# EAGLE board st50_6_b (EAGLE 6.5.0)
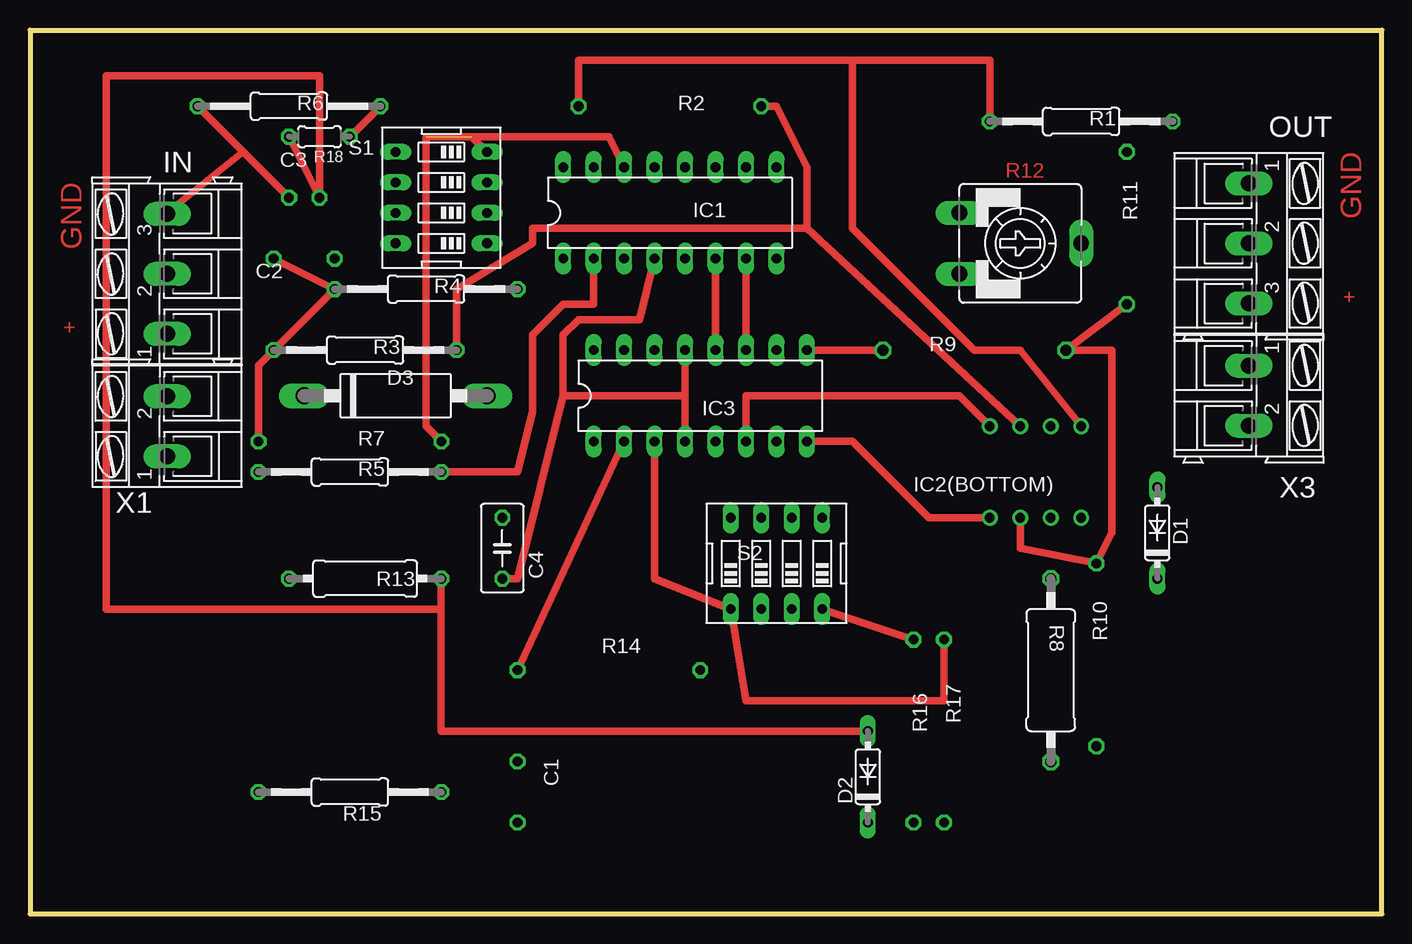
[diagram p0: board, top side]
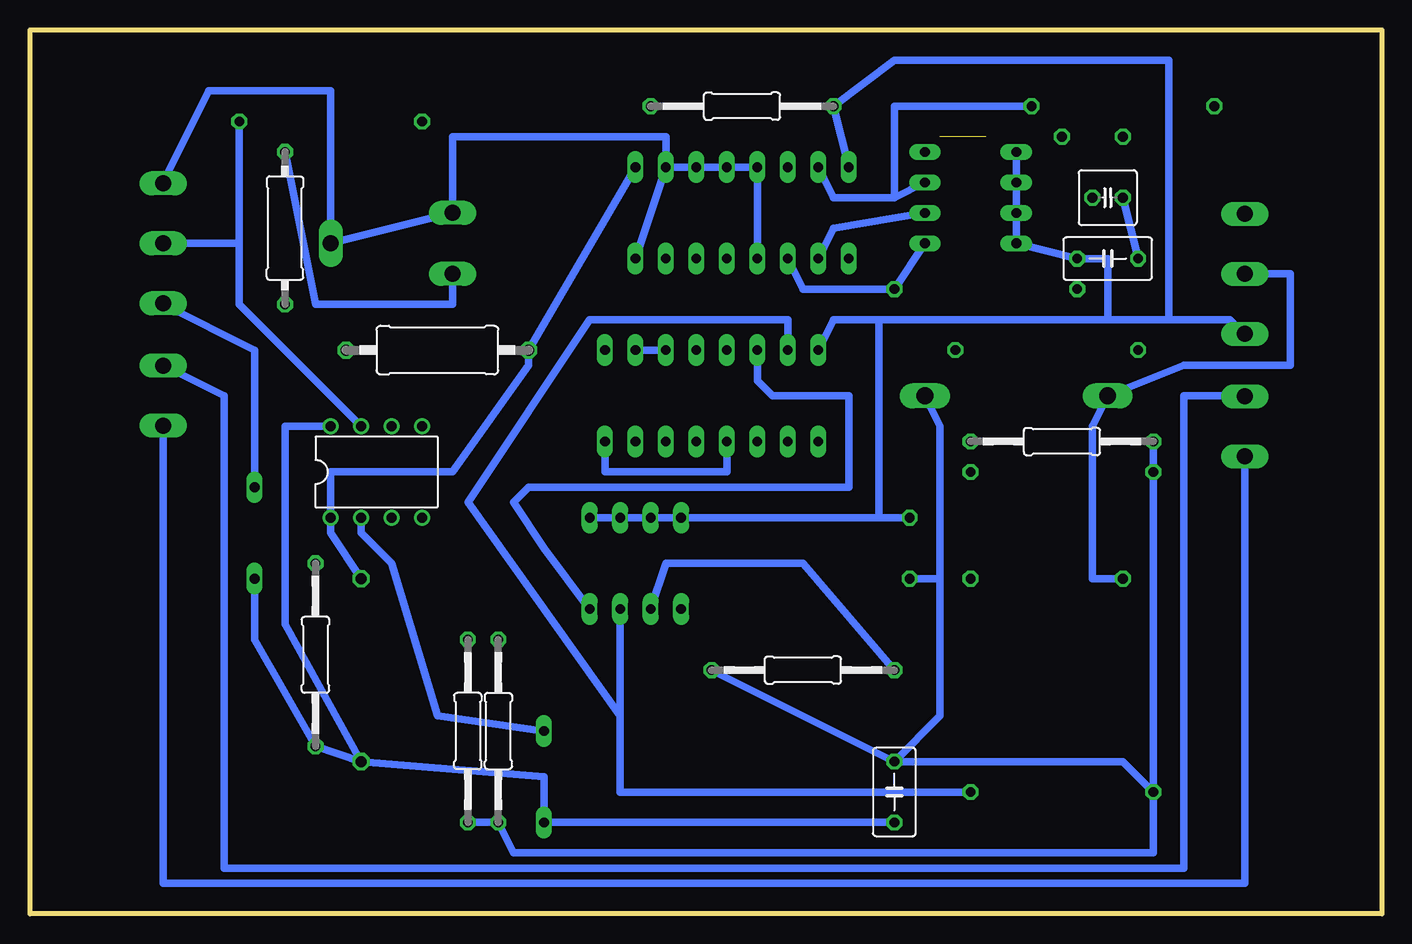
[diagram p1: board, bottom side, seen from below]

Size 112.7 x 73.66 mm. Coordinates in mm from the lower left corner, seen from the top.
Outline: 112.7,73.65 112.7,0 0,0 0,73.65
Outline: 0,73.66 112.7,73.66
Copper layers (1*16): Top 0.035mm / dielectric 1.5mm / Bottom 0.035mm
Design rules "ST50_4 *": minimum track width 0.4mm, minimum drill 24mil, track to track 0.4mm, track to pad 0.4mm, pad to pad 0.4mm, via to via 0.4mm, smd to smd 8mil, copper to edge 40mil, drill to drill 8mil, minimum pad ring 10mil, minimum via ring 8mil, stop-mask expansion 4mil, vias tented up to drill 0mil, thermal gap 10mil
Net classes: 0 default: clearance 0.355 mm

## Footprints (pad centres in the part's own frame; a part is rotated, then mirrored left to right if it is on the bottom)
C050-035X075 = drill 0.813 octagon: 1 -2.54,0; 2 2.54,0
C025-050X050 = drill 0.813 octagon: 1 -1.27,0; 2 1.27,0
DO35-7 = drill 0.813 long: A 3.81,0; C -3.81,0
C1702-15 = drill 1.397 long: A 7.62,0; C -7.62,0
DIL16 = drill 0.813 long: 1 -8.89,-3.81; 2 -6.35,-3.81; 3 -3.81,-3.81; 4 -1.27,-3.81; 5 1.27,-3.81; 6 3.81,-3.81; 7 6.35,-3.81; 8 8.89,-3.81; 9 8.89,3.81; 10 6.35,3.81; 11 3.81,3.81; 12 1.27,3.81; 13 -1.27,3.81; 14 -3.81,3.81; 15 -6.35,3.81; 16 -8.89,3.81
DIL08 = drill 0.813 pad 1.27: 1 -3.81,-3.81; 2 -1.27,-3.81; 3 1.27,-3.81; 4 3.81,-3.81; 5 3.81,3.81; 6 1.27,3.81; 7 -1.27,3.81; 8 -3.81,3.81
AK300/3 = drill 1.321 long: 1 -5.004,0; 2 0,0; 3 5.004,0
0207/15 = drill 0.813 octagon: 1 -7.62,0; 2 7.62,0
0411/15 = drill 0.914 octagon: 1 -7.62,0; 2 7.62,0
0309/12 = drill 0.813 octagon: 1 -6.35,0; 2 6.35,0
CA9V = drill 1.321 long: A -2.54,-5.08; E 2.54,-5.08; S 0,5.08
0204/5 = drill 0.813 octagon: 1 -2.54,0; 2 2.54,0
EDG-04 = drill 0.813 long: 1 -3.81,-3.81; 2 -1.27,-3.81; 3 1.27,-3.81; 4 3.81,-3.81; 5 3.81,3.81; 6 1.27,3.81; 7 -1.27,3.81; 8 -3.81,3.81
AK300/2 = drill 1.321 long: 1 -2.515,0; 2 2.489,0

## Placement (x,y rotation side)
C1  100nF  [C050-035X075]  40.64,10.16 90 bottom
C2  1µF 16V  [C050-035X075]  22.86,54.61 0 bottom
C3  10nF 50V  [C025-050X050]  22.86,59.69 0 bottom
C4  1µF 16V  [C050-035X075]  39.37,30.48 270 top
D1  1N4148DO35-7  [DO35-7]  93.98,31.75 90 top
D2  1N4148DO35-7  [DO35-7]  69.85,11.43 90 top
D3  1N5340  [C1702-15]  30.48,43.18 0 top
IC1  4089N  [DIL16]  53.34,58.42 0 top
IC2(BOTTOM)  LM393N  [DIL08]  83.82,36.83 0 bottom
IC3  4089N  [DIL16]  55.88,43.18 0 top
IN  IN  [AK300/3]  11.43,53.34 90 top
OUT  [AK300/3]  101.6,55.88 270 top
R1  10k  [0207/15]  87.63,66.04 0 top
R2  10k  [0207/15]  53.34,67.31 0 bottom
R3  10k  [0207/15]  27.94,46.99 0 top
R4  10k  [0207/15]  33.02,52.07 0 top
R5  10k  [0207/15]  26.67,36.83 0 top
R6  10k  [0207/15]  21.59,67.31 0 top
R7  10k  [0207/15]  26.67,39.37 0 bottom
R8  4.7k  [0411/15]  85.09,20.32 270 top
R9  1M  [0411/15]  78.74,46.99 0 bottom
R10  10k  [0207/15]  88.9,21.59 90 bottom
R11  1k  [0309/12]  91.44,57.15 270 bottom
R12  10k  [CA9V]  82.55,55.88 270 top
R13  22k  [0309/12]  27.94,27.94 0 top
R14  10k  [0207/15]  48.26,20.32 0 bottom
R15  10k  [0207/15]  26.67,10.16 0 top
R16  10k  [0207/15]  73.66,15.24 270 bottom
R17  10k  [0207/15]  76.2,15.24 90 bottom
R18  2M  [0204/5]  24.13,64.77 180 top
S1  Dip 4  [EDG-04]  34.29,59.69 90 top
S2  Dip 4  [EDG-04]  62.23,29.21 0 top
X1  [AK300/2]  11.43,40.64 90 top
X3  [AK300/2]  101.6,43.18 270 top

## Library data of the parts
C1-C4 R1-R11 R13-R18 = rcl
D1-D3 = diode
IC1 IC3 = 40xx
IC2(BOTTOM) = linear
IN OUT X1 X3 = con-ptr500; OC_FARNELL: unknown; OC_NEWARK: unknown
R12 = pot
S1 S2 = special

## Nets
+8V: C1.1 C2.1 C4.1 D1.C D2.C IC1.16 IC2(BOTTOM).8 IC3.16 IN.1 R1.1 R2.2 R8.2 R10.1 S1.5 S1.6 S1.7 S1.8 S2.5 S2.6 S2.7 S2.8
GND: C1.2 C2.2 C3.2 C4.2 D3.A IC1.4 IC1.8 IC1.10 IC1.11 IC1.12 IC1.13 IC2(BOTTOM).4 IC3.4 IC3.8 IC3.13 IN.3 OUT.1 R3.1 R4.1 R5.1 R6.1 R7.2 R12.A R12.S R14.1 R15.1 R16.2 R17.1
N$1: IC2(BOTTOM).6 R2.1 R3.2
N$2: IC2(BOTTOM).7 OUT.2 R1.2
N$3: IC1.6 IC3.12
N$4: IC1.3 R4.2 S1.1
N$5: IC1.2 R5.2 S1.2
N$6: IC1.15 R6.2 R18.1 S1.3
N$7: IC1.14 R7.1 S1.4
N$9: IC1.9 IC2(BOTTOM).1 IC3.9 R8.1 R9.2
N$10: D1.A OUT.3
N$11: C3.1 D2.A IC2(BOTTOM).2 R13.2 R18.2
N$12: IC2(BOTTOM).3 R9.1 R10.2 R11.2
N$13: R11.1 R12.E
N$14: IC1.7 IC3.10 IC3.11
N$15: IC2(BOTTOM).5 IC3.6
N$16: IC3.3 R17.2 S2.1
N$18: IC3.14 R16.1 S2.4
N$19: IC3.15 R15.2 S2.3
N$20: IC3.2 R14.2 S2.2
N$21: X1.2 X3.1
N$22: X1.1 X3.2
SIGNAL_IN: D3.C IN.2 R13.1

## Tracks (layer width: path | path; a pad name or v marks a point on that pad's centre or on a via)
+8V
  Top 0.61: 68.58,71.12 45.72,71.12 R2.2 | R1.1 80.01,71.12 68.58,71.12 | 68.58,71.12 68.58,57.15 78.74,46.99 82.55,46.99 IC2(BOTTOM).8
  Bottom 0.4: 11.43,48.26 IN.1
  Bottom 0.61: C1.1 D2.C 69.85,11.43 R8.2 | D1.C 93.98,22.86 R10.1 R8.2 | IC2(BOTTOM).8 91.44,40.64 91.44,24.13 R8.2 | IC1.16 R2.2 40.64,71.12 17.78,71.12 17.78,49.53 | 17.78,49.53 22.86,49.53 | 22.86,49.53 41.91,49.53 | 41.91,49.53 45.72,49.53 IC3.16 | 11.43,48.26 12.7,49.53 17.78,49.53 | S1.5 S1.6 S1.7 S1.8 C2.1 22.86,54.61 22.86,49.53 | S2.5 S2.6 S2.7 S2.8 41.91,33.02 | 41.91,33.02 C4.1 | 41.91,33.02 41.91,49.53
GND
  Top 0.4: 11.43,58.42 IN.3
  Top 0.61: R6.1 17.78,63.5 | 17.78,63.5 C3.2 | C2.2 R4.1 R3.1 19.05,45.72 R7.2 | 44.45,43.18 54.61,43.18 | 54.61,43.18 IC3.4 | 44.45,43.18 40.64,27.94 C4.2 | IC3.13 54.61,43.18 | IC1.4 50.8,49.53 45.72,49.53 44.45,48.26 44.45,43.18 | IC2(BOTTOM).4 74.93,33.02 68.58,39.37 IC3.8 | 17.78,63.5 11.43,58.42
  Bottom 0.4: 101.6,60.96 OUT.1
  Bottom 0.61: C2.2 C3.2 | IC1.4 IC1.13 IC1.12 IC1.11 IC1.10 | IC1.10 IC1.8 | 36.83,27.94 36.83,16.51 C1.2 | IC1.10 59.69,64.77 77.47,64.77 R12.A R12.S 87.63,68.58 97.79,68.58 101.6,60.96 | C1.2 21.59,12.7 R15.1 | R15.1 R5.1 R7.2 | R17.1 R16.2 | C1.2 R14.1 | R16.2 72.39,5.08 19.05,5.08 R15.1 | 74.93,7.62 R16.2 | D3.A 36.83,40.64 36.83,27.94 | 36.83,27.94 C4.2 | IC3.8 64.77,36.83 54.61,36.83 IC3.4
N$1
  Top 0.61: R2.1 62.23,67.31 64.77,62.23 64.77,57.15 | 64.77,57.15 41.91,57.15 41.91,55.88 35.56,52.07 R3.2 | IC2(BOTTOM).6 64.77,57.15
N$2
  Bottom 0.61: IC2(BOTTOM).7 95.25,50.8 95.25,55.88 | 95.25,55.88 R1.2 | 95.25,55.88 OUT.2
N$3
  Top 0.61: IC1.6 IC3.12
N$4
  Bottom 0.61: S1.1 R4.2 48.26,52.07 IC1.3
N$5
  Top 0.61: IC1.2 46.99,50.8 44.45,50.8 41.91,48.26 41.91,41.91 40.64,36.83 R5.2
  Bottom 0.61: IC1.2 45.72,57.15 S1.2
N$6
  Top 0.61: R18.1 R6.2 27.94,67.31
  Bottom 0.61: 40.64,59.69 S1.3 | R6.2 40.64,67.31 40.64,59.69 | IC1.15 45.72,59.69 40.64,59.69
N$7  (1 unrouted)
  Top 0.61: IC1.14 48.26,64.77 33.02,64.77 33.02,40.64 R7.1 | S1.4 36.83,64.77
N$9
  Top 0.61: IC3.9 R9.2
  Bottom 0.61: IC1.9 R9.2 71.12,45.72 77.47,36.83 87.63,36.83 IC2(BOTTOM).1 87.63,31.75 R8.1
N$10
  Bottom 0.4: 101.6,50.8 OUT.3
  Bottom 0.61: D1.A 93.98,46.99 101.6,50.8
N$11
  Top 0.61: 34.29,25.4 6.35,25.4 6.35,69.85 24.13,69.85 C3.1 R18.2 | R13.2 34.29,25.4 | 34.29,25.4 34.29,15.24 D2.A
  Bottom 0.61: D2.A 78.74,16.51 82.55,29.21 85.09,31.75 IC2(BOTTOM).2
N$12
  Top 0.61: R11.2 R9.1 90.17,46.99 90.17,31.75 R10.2 82.55,30.48 IC2(BOTTOM).3
N$13
  Bottom 0.61: R12.E 77.47,50.8 88.9,50.8 R11.1
N$14
  Top 0.61: IC3.11 IC1.7
  Bottom 0.61: IC3.10 IC3.11
N$15
  Top 0.61: IC3.6 59.69,43.18 77.47,43.18 IC2(BOTTOM).5
N$16
  Top 0.61: IC3.3 52.07,27.94 S2.1 59.69,17.78 76.2,17.78 R17.2
N$18
  Top 0.61: R16.1 S2.4
  Bottom 0.61: IC3.14 52.07,44.45 50.8,43.18 44.45,43.18 44.45,35.56 71.12,35.56 72.39,34.29 69.85,30.48 S2.4
N$19
  Bottom 0.61: R15.2 63.5,10.16 63.5,16.51 | IC3.15 49.53,49.53 66.04,49.53 76.2,34.29 63.5,16.51 | S2.3 63.5,16.51
N$20
  Top 0.61: IC3.2 R14.2
  Bottom 0.61: S2.2 59.69,29.21 48.26,29.21 R14.2
N$21
  Bottom 0.4: 101.6,45.72 X3.1 | 11.43,43.18 X1.2
  Bottom 0.61: 11.43,43.18 16.51,43.18 16.51,3.81 96.52,3.81 96.52,43.18 101.6,45.72
N$22
  Bottom 0.4: 11.43,38.1 X1.1
  Bottom 0.61: 11.43,38.1 11.43,2.54 101.6,2.54 X3.2
SIGNAL_IN
  Bottom 0.61: R13.1 24.13,27.94 24.13,40.64 D3.C 16.51,45.72 7.62,45.72 7.62,53.34 IN.2

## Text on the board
Top: GND | GND | + | +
